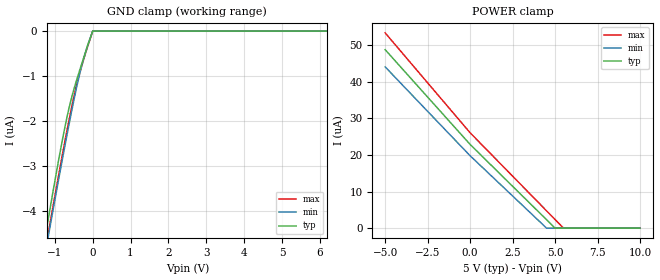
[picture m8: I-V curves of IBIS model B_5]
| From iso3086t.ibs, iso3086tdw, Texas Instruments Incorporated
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|   B_5 Model
[Model]   B_5
Model_type   Input
|Signals   B   negative pin
|Rref = 27   Note: 54 Ohm differential load;
Vinl   = 1.5V
Vinh   = 3.5V
|Rref_Diff   = 96kOhms   |Input Diff resistance
|Cref_Diff   = 7pF   |Input Diff capacitance
|Vdiff can be <= -200mV or >=-100mV and Common mode can be betweem -7V to 12V
|C_comp   typ   min   max
|   (Nom PVT)   (Slow PVT)   (Fast PVT)
C_comp   1.0130724pF  1.0130723pF  1.0130724pF
[Model Spec]
Vinl   1.5V   1.35V   1.65V
Vinh   3.5V   3.15V   3.85V
[Voltage Range]   5   4.5   5.5
[Temperature Range]   40   125   -40
[Power Clamp Reference]   5   4.5   5.5
[GND Clamp Reference]   0   0   0
[GND Clamp]
|   Voltage   I(typ)   I(min)   I(max)
-5V       -24.05uA   -23.38uA   -24.97uA
-1.295V   -4.787uA   -5.146uA   -5.082uA
-1.183V   -4.23uA    -4.617uA   -4.539uA
-1.16V    -4.119uA   -4.512uA   -4.431uA
-1.145V   -4.046uA   -4.442uA   -4.36uA
-792.5mV  -2.391uA   -2.821uA   -2.714uA
-605mV    -1.645uA   -1.995uA   -1.896uA
-440mV    -1.136uA   -1.317uA   -1.255uA
-290mV    -734.3nA   -776.7nA   -780.4nA
-140mV    -341.8nA   -335.3nA   -361.7nA
2.5mV     0A         0A         0A
10V       0A         0A         0A
[POWER Clamp]
|   Voltage   I(typ)   I(min)   I(max)
-5V       48.71uA    44.02uA    53.3uA
2.5mV     22.84uA    19.75uA    26.02uA
4.503V    2.294uA    0A         4.721uA
5.005V    0A         0A         2.343uA
5.5V      0A         0A         0A
10V       0A         0A         0A
